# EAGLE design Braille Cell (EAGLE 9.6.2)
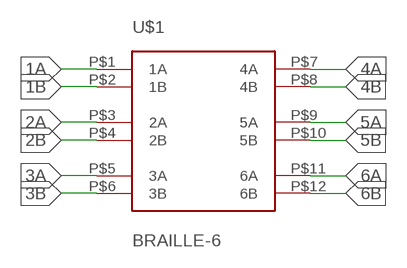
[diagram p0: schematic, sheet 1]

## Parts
U$1  BRAILLE-6  [BRAILLE-6]

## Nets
1A: U$1.P$1(1A)
1B: U$1.P$2(1B)
2A: U$1.P$3(2A)
2B: U$1.P$4(2B)
3A: U$1.P$5(3A)
3B: U$1.P$6(3B)
4A: U$1.P$7(4A)
4B: U$1.P$8(4B)
5A: U$1.P$9(5A)
5B: U$1.P$10(5B)
6A: U$1.P$11(6A)
6B: U$1.P$12(6B)

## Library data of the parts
U$1 = Braille Cell:BRAILLE-6

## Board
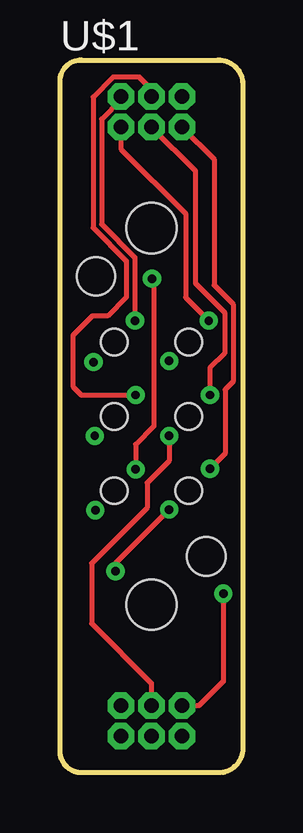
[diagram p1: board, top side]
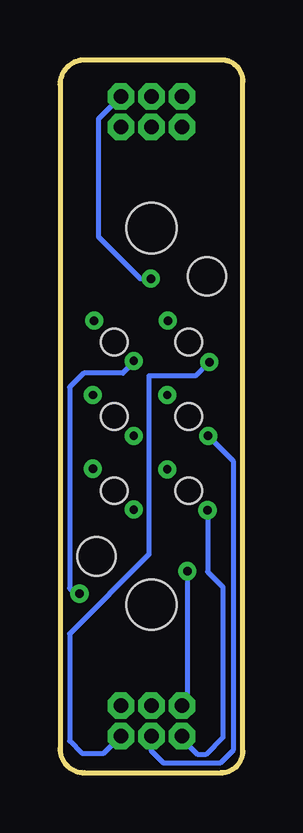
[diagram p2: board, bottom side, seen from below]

Size 7.62 x 29.72 mm. Coordinates in mm from the lower left corner, seen from the top.
Outline: 7.62,28.7 7.62,1.02 arc-90 6.6,0 0.91,0 arc-90 0,0.91 0,28.83 arc-90 0.89,29.72 6.58,29.72 arc-90 7.62,28.7
Copper layers (1*16): Top 0.035mm / dielectric 1.5mm / Bottom 0.035mm
Design rules "default *": minimum track width 6mil, minimum drill 0.35mm, track to track 6mil, track to pad 6mil, pad to pad 6mil, via to via 6mil, smd to smd 6mil, copper to edge 0.2mm, drill to drill 6mil, minimum pad ring 10mil, minimum via ring 8mil, stop-mask expansion 4mil, vias tented up to drill 0mil, thermal gap 10mil
Holes 1.1 mm at 2.26,17.96 5.36,17.96 2.26,14.86 5.36,14.86 2.26,11.76 5.36,11.76
Holes 2.1 mm at 3.81,22.71 3.81,7.01
Holes 1.6 mm at 1.5,20.7 6.1,9.02

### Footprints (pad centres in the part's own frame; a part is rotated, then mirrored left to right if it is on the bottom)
BRAILLE-6 = drill 0.6 octagon: P$1 -1.27,13.335; P$2 1.27,-13.335; P$3 0,13.335; P$4 0,-13.335; P$5 1.27,13.335; P$6 -1.27,-13.335; P$7 -1.27,12.065; P$8 1.27,-12.065; P$9 0,12.065; P$10 0,-12.065; P$11 1.27,12.065; P$12 -1.27,-12.065

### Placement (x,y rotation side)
U$1  3.81,14.86 0 top

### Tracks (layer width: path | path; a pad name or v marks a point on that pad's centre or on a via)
1A  (via drill 0.35)
  Top 0.203: U$1.P$1 2.54,28.07 1.73,27.26 1.73,22.87 3.12,21.48 v3.12,18.85
1B  (via drill 0.35)
  Bottom 0.203: v1.4,17.12 1.41,17.12 1.98,16.55 3.91,16.55 3.91,9.1 7.22,5.79 7.22,1.32 6.71,0.81 5.79,0.81 U$1.P$2
2A  (via drill 0.35)
  Top 0.203: U$1.P$3 3.81,28.5 3.31,29 2.21,29 1.38,28.17 1.38,22.73 2.77,21.34 2.77,19.84 1.98,19.05 1.35,19.05 0.53,18.24 0.53,16.1 0.89,15.75 v3.15,15.75
2B  (via drill 0.35)
  Bottom 0.203: v1.45,14.05 0.4,13 0.4,0.94 0.94,0.4 3.3,0.4 3.81,0.91 U$1.P$4
3A  (via drill 0.35)
  Top 0.203: U$1.P$5 5.21,28.19 | v3.84,20.6 3.91,20.52 3.91,14.45 3.15,13.69 v3.15,12.65
  Bottom 0.203: 3.58,20.6 v3.84,20.6 4.27,20.6 6.02,22.35 6.02,27.25 U$1.P$5
3B  (via drill 0.35)
  Bottom 0.203: v1.47,10.95 1.47,8.38 0.84,7.75 0.84,1.47 1.55,0.76 1.88,0.76 2.54,1.42 U$1.P$6
4A  (via drill 0.35)
  Top 0.203: U$1.P$7 2.54,26.01 5.23,23.32 5.23,19.81 v6.2,18.85
4B  (via drill 0.35)
  Top 0.203: v6.81,7.47 6.81,3.81 5.79,2.79 U$1.P$8
  Bottom 0.203: v6.81,7.47 6.99,7.47 7.22,7.7 7.22,16.07 6.63,16.66 5,16.66 4.55,17.12 v4.55,17.17
5A  (via drill 0.35)
  Top 0.203: U$1.P$9 5.64,25.09 5.64,20.41 6.86,19.19 6.86,17.49 6.25,16.88 v6.25,15.75
5B  (via drill 0.35)
  Top 0.203: v4.55,14.05 4.55,13 3.63,12.09 3.63,11.05 1.32,8.74 1.32,6.22 3.81,3.73 U$1.P$10
6A  (via drill 0.35)
  Top 0.203: U$1.P$11 6.43,25.58 6.43,20.32 7.21,19.54 7.21,16.3 6.88,15.98 6.88,13.31 v6.25,12.68
6B  (via drill 0.35)
  Top 0.203: v4.55,10.97 2.31,8.74 v2.31,8.41
  Bottom 0.203: v2.31,8.41 2.31,3.02 U$1.P$12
